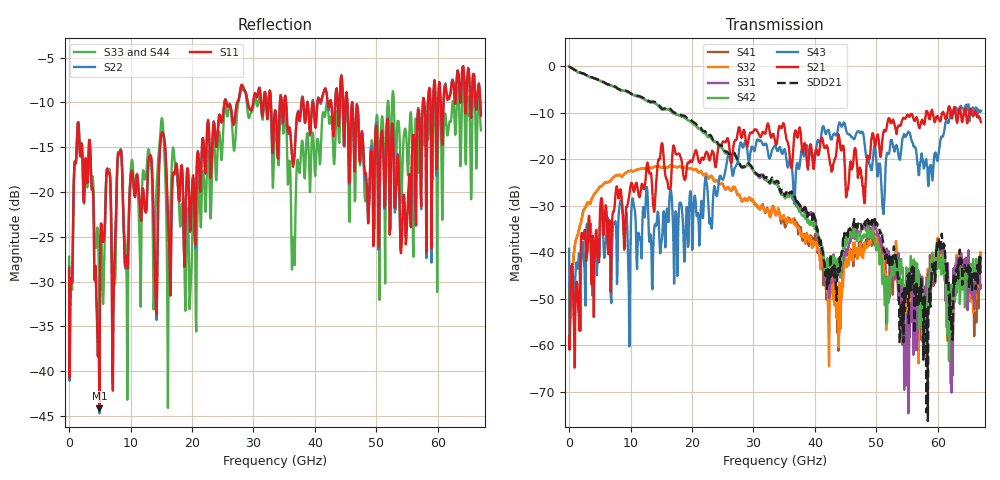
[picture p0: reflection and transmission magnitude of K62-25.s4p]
!Agilent Technologies,N5247A,US50470101,A.10.25.02
!Agilent N5247A: A.10.25.02
!Date: Tuesday, May 12, 2015 13:41:33
!Correction: Sdd11(Full 4 Port(1,2,3,4))
!Sdc11(Full 4 Port(1,2,3,4))
!Sdd12(Full 4 Port(1,2,3,4))
!Sdc12(Full 4 Port(1,2,3,4))
!Scd11(Full 4 Port(1,2,3,4))
!Scc11(Full 4 Port(1,2,3,4))
!Scd12(Full 4 Port(1,2,3,4))
!Scc12(Full 4 Port(1,2,3,4))
!Sdd21(Full 4 Port(1,2,3,4))
!Sdc21(Full 4 Port(1,2,3,4))
!Sdd22(Full 4 Port(1,2,3,4))
!Sdc22(Full 4 Port(1,2,3,4))
!Scd21(Full 4 Port(1,2,3,4))
!Scc21(Full 4 Port(1,2,3,4))
!Scd22(Full 4 Port(1,2,3,4))
!Scc22(Full 4 Port(1,2,3,4))
!Balanced Topology: BBAL
!S4P File: Measurements: <Sdd11,Sdc11,Sdd12,Sdc12>,
!<Scd11,Scc11,Scd12,Scc12>,
!<Sdd21,Sdc21,Sdd22,Sdc22>,
!<Scd21,Scc21,Scd22,Scc22>:
# Hz S  dB  R 50
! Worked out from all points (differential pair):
!   801 points, 10 MHz to 67 GHz, reference 50 ohm
!   strongest paths, dB at 10 MHz, 16.76 GHz, 33.51 GHz, 50.25 GHz, 67 GHz:
!     S21: -58.2, -20.2, -16.0, -14.7, -12.0
!     S43: -39.3, -29.2, -17.1, -23.4, -9.6
!     S42: 0.0, -9.9, -25.0, -38.8, -41.3
!     S31: 0.0, -9.9, -25.3, -36.4, -47.2
!     S32: -47.7, -21.5, -31.5, -37.9, -43.7
!     S41: -46.7, -21.5, -31.1, -37.8, -42.7
!   taken as a pair (ports 2,1 in; 4,3 out), SDD21 dB: 0.0, -9.6, -25.0, -34.4, -40.9
!   lowest |S11| = -44.2 dB at 4.951 GHz (marker M1), VSWR 1.01, Z = 50.6 - j0.0703 ohm
!   |S11| at or under -10 dB: start of sweep to 25.29 GHz; 35.32 GHz to 37.83 GHz (2.512 GHz wide, 6.87 % of centre); 46.07 GHz to 57.57 GHz (11.5 GHz wide, 22.2 % of centre)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
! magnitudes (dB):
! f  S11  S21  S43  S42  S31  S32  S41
! 10 MHz  -28.5  -58.2  -39.3  0.0  0.0  -47.7  -46.7
! 1.685 GHz  -14.6  -56.9  -41.1  -1.3  -1.3  -34.9  -34.9
! 4.951 GHz  -44.2  -35.4  -41.1  -3.1  -3.1  -26.1  -26.1
! 43.8 GHz  -11.9  -14.6  -13.0  -42.9  -44.9  -49.2  -61.2
! 49.67 GHz  -18.7  -16.1  -17.2  -37.0  -35.0  -36.9  -38.4
! 55.03 GHz  -22.6  -10.4  -14.5  -44.8  -53.2  -57.6  -52.0
! 67 GHz  -11.5  -12.0  -9.6  -41.3  -47.2  -43.7  -42.7
